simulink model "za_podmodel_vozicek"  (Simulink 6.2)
settings: Solver=ode45  StartTime=0.0  StopTime=10.0  RelTol=1e-3
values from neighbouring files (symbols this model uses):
  k1 = KK(1)    [ch8_d.m]    (also in set_x4a.m = 1; za_podmodel_voz.m = 1; auto_param.m = 7500; auto_param_opt.m = 15000)
  k2 = KK(2)    [ch8_d.m]    (also in set_x4a.m = 2; za_podmodel_voz.m = 2; auto_param.m = 150000; auto_param_opt.m = 150000)
  m1 = 10    [ex12_2st.m]    (also in set_x4a.m = 1; za_podmodel_voz.m = 1; Naloga31.m = 500)
  v10 = 0    [set_x4a.m]    (also in za_podmodel_voz.m)
  x10 = 1    [set_x4a.m]    (also in za_podmodel_voz.m)

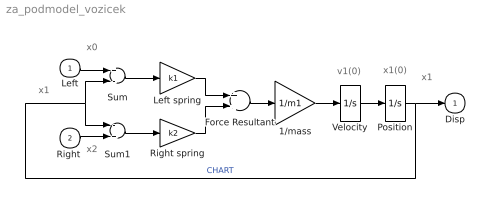
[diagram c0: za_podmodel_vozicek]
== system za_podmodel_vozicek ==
  note: x0
  note: x1
  note: x1
  note: x2
  note: v1(0)
  note: x1(0)
  Left : Inport  Port=1  LatchInput=off
  "Right " : Inport  Port=2  LatchInput=off
  1/mass : Gain  Gain=1/m1
  Force Resultant : Sum
  Left spring : Gain  Gain=k1
  Position : Integrator  InitialCondition=x10
  Right spring : Gain  Gain=k2
  Sum : Sum  Inputs=+-
  Sum1 : Sum  Inputs=-+
  Velocity : Integrator  InitialCondition=v10
  Disp : Outport  InitialOutput=0
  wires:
  Position/1 -> Sum1/1, Sum/2, Disp/1  "CHART"
  Velocity/1 -> Position/1
  1/mass/1 -> Velocity/1
  Force Resultant/1 -> 1/mass/1
  Right spring/1 -> Force Resultant/2
  Left spring/1 -> Force Resultant/1
  Sum/1 -> Left spring/1
  Sum1/1 -> Right spring/1
  "Right "/1 -> Sum1/2
  Left/1 -> Sum/1
